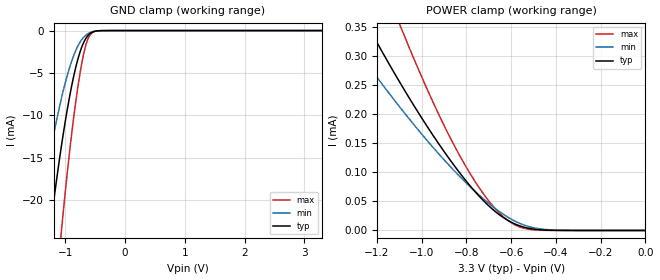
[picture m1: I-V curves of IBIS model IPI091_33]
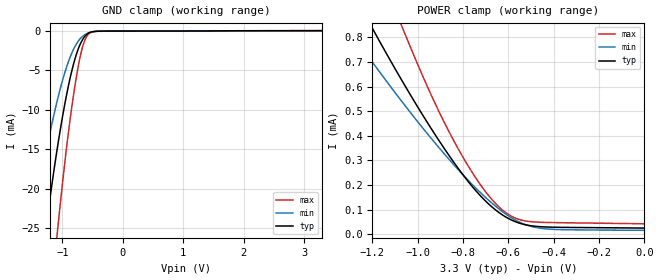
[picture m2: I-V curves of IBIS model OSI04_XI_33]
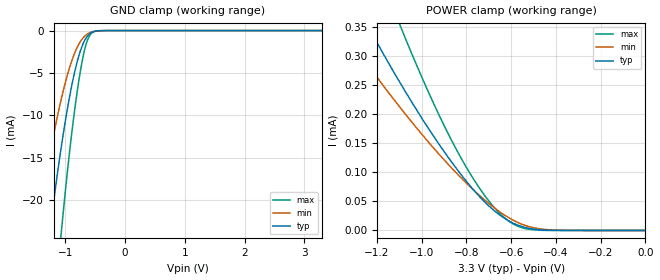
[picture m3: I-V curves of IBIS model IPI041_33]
| TEXAS INSTRUMENTS INCORPORATED
| Connectivity Solutions Group
| IBIS Model of TL16C550DRHB_3.3V
| 550D_RHB_3.3V
| This file contains package information for the following:
|  RHB 32-pin (QFN) package as [Component] 550DRHB_3.3V
| This device can be powered at the following Vccs:
|  3.3 Volt Vcc
| This file provides unique models under the [Model Selector] for each Vcc.
| For operation at a specific Vcc, select the appropriate model after each
| [Model Selector] keyword.
[IBIS Ver]   3.2
[Comment char]  |_char
[File Name]   550D_RHB_3.3V.ibs
[File Rev]   1 | a
[Date]   January 5, 2009
[Source]   Data created from TI-SPICE simulations at TI-CONN.
[Notes]   The following is an IBIS list for the 550D_RHB_3.3V.
   Please contact s-ly@ti.com with questions and
   comments concerning CONN IBIS models.
[Disclaimer] Property of Texas Instruments Incorporated.  Unauthorized
   reproduction and/or distribution is strictly prohibited.
   This product is protected under copyright law.
   Created  2003, (C) Copyright  2003, Texas Instruments
   Incorporated, All Rights Reserved
   UNLESS THERE IS A SIGNED, WRITTEN AGREEMENT TO THE
   CONTRARY, TEXAS INSTRUMENTS (TI) IS PROVIDING THE IBIS
   MODELS  AND WITHOUT ANY WARRANTY, EXPRESSED OR
   IMPLIED.  TI assumes no liability for:
   1) the accuracy of the IBIS models provided to your
   company;
   2) the proper functioning of these IBIS Models in your
   design or for any resulting applications; or
   3) infringement of patents, copyrights or intellectual
   property rights resulting from your use of these IBIS
   models.
   TI provides IBIS Models as a service to our customers.
   You and your company shall not distribute, sell or give
   these models to anyone else without prior written
   permission from TI.
   TI reserves the right to make changes to our products or
   to discontinue any semiconductor product or service
   without notice, and advises our customers to obtain the
   latest version of relevant information to verify, before
   placing orders, that the information being relied on is
   current.
   Please be aware that your receipt and use of the IBIS
   information provided shall serve as acceptance of these
   terms and conditions.  If you do not accept these terms,
   you should return or destroy the IBIS models and any
   other accompanying information immediately.
| Component 550D_3.3V_RHB 32-pin QFN
[Component]   550D_RHB_3.3V
[Manufacturer]   Texas Instruments, Inc.
[Package]
|   typ   min   max
R_pkg   4.900e-04   4.900e-04   4.900e-04
L_pkg   1.009e-10   0.683e-10   1.336e-10
C_pkg   2.424e-14   1.463e-14   3.850e-14
[Pin]   signal_name   model_name   R_pin   L_pin   C_pin
1   D4   IPI04_OPJ43   4.900e-04   1.347e-10   8.118e-14
2   NC   NC   4.900e-04   1.284e-10   9.657e-14
3   D5   IPI04_OPJ43   4.900e-04   1.275e-10   9.662e-14
4   D6   IPI04_OPJ43   4.900e-04   1.273e-10   9.663e-14
5   D7   IPI04_OPJ43   4.900e-04   1.273e-10   9.663e-14
6   SIN   IPI041   4.900e-04   1.275e-10   9.661e-14
7   SOUT   OPJ430   4.900e-04   1.285e-10   9.656e-14
8   CS2B   IPI041   4.900e-04   1.347e-10   8.119e-14
9   NC   NC   4.900e-04   1.347e-10   8.118e-14
10   XIN   OSI04_XI   4.900e-04   1.284e-10   9.657e-14
11   XOUT   OSI04   4.900e-04   1.275e-10   9.662e-14
12   WR1B   IPI041   4.900e-04   1.273e-10   9.663e-14
13   VSS   GND   4.900e-04   1.273e-10   9.663e-14
14   RD1B   IPI041   4.900e-04   1.275e-10   9.660e-14
15   NC   NC   4.900e-04   1.285e-10   9.653e-14
16   NC   NC   4.900e-04   1.348e-10   8.116e-14
17   A2   IPI041   4.900e-04   1.348e-10   8.117e-14
18   A1   IPI041   4.900e-04   1.285e-10   9.656e-14
19   A0   IPI041   4.900e-04   1.275e-10   9.661e-14
20   INTRPT   OPJ430   4.900e-04   1.273e-10   9.662e-14
21   RTSB   OPJ430   4.900e-04   1.273e-10   9.662e-14
22   DTRB   OPJ430   4.900e-04   1.275e-10   9.663e-14
23   MR   IPI091   4.900e-04   1.284e-10   9.657e-14
24   CTSB   IPI041   4.900e-04   1.347e-10   8.117e-14
25   DSRB   IPI041   4.900e-04   1.348e-10   8.117e-14
26   DCDB   IPI041   4.900e-04   1.285e-10   9.656e-14
27   RIB   IPI041   4.900e-04   1.275e-10   9.662e-14
28   VCC   POWER   4.900e-04   1.273e-10   9.663e-14
29   D0   IPI04_OPJ43   4.900e-04   1.273e-10   9.662e-14
30   D1   IPI04_OPJ43   4.900e-04   1.275e-10   9.663e-14
31   D2   IPI04_OPJ43   4.900e-04   1.284e-10   9.657e-14
32   D3   IPI04_OPJ43   4.900e-04   1.348e-10   8.116e-14
| Model IPI091
[Model Selector]   IPI091
IPI091_33   3.3 volt Vcc
| Model OSI04_XI
[Model Selector]   OSI04_XI
OSI04_XI_33   3.3 volt Vcc
| Model IPI041
[Model Selector]   IPI041
IPI041_33   3.3 volt Vcc
| Model IPI04_OPJ43
[Model Selector]   IPI04_OPJ43
IPI04_OPJ43_33   3.3 volt Vcc
| Model OPJ430
[Model Selector]   OPJ430
OPJ430_33   3.3 volt Vcc
| Model OSI04
[Model Selector]   OSI04
OSI04_33   3.3 volt Vcc
| Models and submodels in the file (6): IPI091_33 (Input), OSI04_XI_33 (Input), IPI041_33 (Input), IPI04_OPJ43_33 (I/O), OPJ430_33 (3-state), OSI04_33 (3-state)
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[Model]   IPI091_33
Model_type  Input
Vinl = 0
Vinh = 3.3
| variable   typ   min   max
C_comp   1.07pF   0.95pF   1.20pF
[Temperature Range]   40   125   -40
| Ambient temperature   25   110   -40
[Voltage range]   3.3   3   3.6
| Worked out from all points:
|   GND clamp passes 1 mA (typ) near -0.66 V on its own axis
|   POWER clamp passes 1 mA (typ) near -2.03 V on its own axis
[GND Clamp]
| IPI091_33
|   Voltage   I(typ)   I(min)   I(max)
-3.3V     -184.1mA   -131.7mA   -253.5mA
-1.485V   -37.43mA   -23.94mA   -59.12mA
-1.28V    -24.78mA   -15.34mA   -40.66mA
-1.25V    -23.07mA   -14.2mA    -38.11mA
-1.075V   -13.97mA   -8.224mA   -24.19mA
-1.06V    -13.26mA   -7.774mA   -23.08mA
-940mV    -8.152mA   -4.58mA    -14.87mA
-805mV    -3.718mA   -2.005mA   -7.28mA
-700mV    -1.488mA   -825uA     -2.909mA
-600mV    -421.4uA   -273uA     -659.6uA
-400mV    -8.531uA   -12.92uA   -6.748uA
3.3V      251.6pA    69.15nA    65.83pA
[POWER Clamp]
| IPI091_33
|   Voltage   I(typ)   I(min)   I(max)
-3.3V     2.289mA    1.713mA    3.253mA
-1.35V    432uA      344.6uA    613.8uA
-1.225V   341.4uA    277.2uA    481uA
-1.11V    263.3uA    218.6uA    366.4uA
-1.075V   240.6uA    201.5uA    333.1uA
-930mV    152.9uA    134.7uA    205.1uA
-805mV    87.01uA    83.43uA    112uA
-700mV    42.42uA    46.59uA    50.87uA
-620mV    18.66uA    24.18uA    18.85uA
-540mV    5.375uA    9.01uA     3.55uA
-445mV    638.3nA    1.643uA    187.2nA
-47.99fV  251.6pA    2.2nA      73.1pA
[Model]   OSI04_XI_33
Model_type  Input
Vinl = 0
Vinh = 3.3
| variable   typ   min   max
C_comp   1.85pF   1.15pF   2.42pF
[Temperature Range]   40   125   -40
| Ambient temperature   25   110   -40
[Voltage range]   3.3   3   3.6
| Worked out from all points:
|   GND clamp passes 1 mA (typ) near -0.66 V on its own axis
|   POWER clamp passes 1 mA (typ) near -1.30 V on its own axis
[GND Clamp]
| OSI04_XI_33
|   Voltage   I(typ)   I(min)   I(max)
-3.3V     -187.4mA   -133.6mA   -258.6mA
-1.52V    -40.73mA   -26.12mA   -63.96mA
-1.48V    -38.05mA   -24.28mA   -60.12mA
-1.275V   -25.2mA    -15.59mA   -41.32mA
-1.095V   -15.43mA   -9.17mA    -26.46mA
-1.07V    -14.21mA   -8.387mA   -24.55mA
-935mV    -8.294mA   -4.704mA   -15.09mA
-800mV    -3.791mA   -2.104mA   -7.36mA
-695mV    -1.529mA   -912.1uA   -2.917mA
-600mV    -479.4uA   -361uA     -744.5uA
-390mV    -35.35uA   -32.95uA   -52.71uA
3.3V      25.17uA    17.8uA     39.06uA
[POWER Clamp]
| OSI04_XI_33
|   Voltage   I(typ)   I(min)   I(max)
-3.3V     5.294mA    3.984mA    7.572mA
-1.3V     1.007mA    827.6uA    1.402mA
-1.195V   827.7uA    692.7uA    1.14mA
-1.075V   632.4uA    545.1uA    855.7uA
-1.04V    577.7uA    503.5uA    776.7uA
-915mV    392.6uA    361.2uA    514.8uA
-815mV    259.4uA    256uA      336.3uA
-720mV    152.9uA    166.1uA    196.6uA
-625mV    77.8uA     91.06uA    97.45uA
-555mV    46.18uA    50.98uA    60.77uA
-455mV    30.55uA    24.01uA    48.59uA
-47.99fV  25.17uA    16.02uA    42.63uA
[Model]   IPI041_33
Model_type  Input
Vinl = 0
Vinh = 3.3
| variable   typ   min   max
C_comp   1.08pF   0.95pF   1.21pF
[Temperature Range]   40   125   -40
| Ambient temperature   25   110   -40
[Voltage range]   3.3   3   3.6
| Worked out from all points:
|   GND clamp passes 1 mA (typ) near -0.66 V on its own axis
|   POWER clamp passes 1 mA (typ) near -2.03 V on its own axis
[GND Clamp]
| IPI041_33
|   Voltage   I(typ)   I(min)   I(max)
-3.3V     -184.1mA   -131.7mA   -253.5mA
-1.485V   -37.43mA   -23.94mA   -59.12mA
-1.28V    -24.78mA   -15.34mA   -40.66mA
-1.25V    -23.07mA   -14.2mA    -38.11mA
-1.075V   -13.97mA   -8.224mA   -24.19mA
-1.06V    -13.26mA   -7.774mA   -23.08mA
-940mV    -8.152mA   -4.58mA    -14.87mA
-805mV    -3.718mA   -2.005mA   -7.28mA
-700mV    -1.488mA   -825uA     -2.909mA
-600mV    -421.4uA   -273uA     -659.6uA
-400mV    -8.531uA   -12.92uA   -6.748uA
3.3V      251.6pA    69.15nA    65.83pA
[POWER Clamp]
| IPI041_33
|   Voltage   I(typ)   I(min)   I(max)
-3.3V     2.289mA    1.713mA    3.253mA
-1.35V    432uA      344.6uA    613.8uA
-1.225V   341.4uA    277.2uA    481uA
-1.11V    263.3uA    218.6uA    366.4uA
-1.075V   240.6uA    201.5uA    333.1uA
-930mV    152.9uA    134.7uA    205.1uA
-805mV    87.01uA    83.43uA    112uA
-700mV    42.42uA    46.59uA    50.87uA
-620mV    18.66uA    24.18uA    18.85uA
-540mV    5.375uA    9.01uA     3.55uA
-445mV    638.3nA    1.643uA    187.2nA
-47.99fV  251.6pA    2.2nA      73.1pA
